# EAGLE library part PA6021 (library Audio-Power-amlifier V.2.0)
The PA6021 is a stereo audio power amplifier that drives 2 W/channel of continuous RMS power into a 4-Ω load when utilizing a heat sink. Advanced dc volume control minimizes external components and allows BTL (speaker) volume control and SE (headphone) volume control.
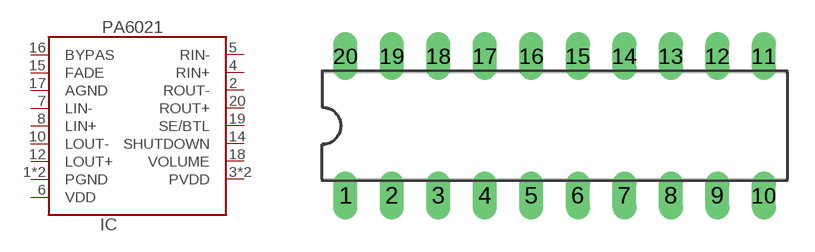
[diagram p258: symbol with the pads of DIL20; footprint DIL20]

Designator prefix IC

## PA6021  [DIL20]
1  PGND  pwr
2  ROUT-  out
3  PVDD  pwr
4  RIN+  in
5  RIN-  in
6  VDD  pwr
7  LIN-  in
8  LIN+  in
9  PVDD  pwr
10  LOUT-  out
11  PGND  pwr
12  LOUT+  out
14  SHUTDOWN  in
15  FADE  in
16  BYPAS  in
17  AGND  pwr
18  VOLUME  in
19  SE/BTL  in
20  ROUT+  out

## Footprint DIL20 (pad centres in mm)
Dual In Line Package
drill 0.813 long: 1 -11.43,-3.81; 2 -8.89,-3.81; 3 -6.35,-3.81; 4 -3.81,-3.81; 5 -1.27,-3.81; 6 1.27,-3.81; 7 3.81,-3.81; 8 6.35,-3.81; 9 8.89,-3.81; 10 11.43,-3.81; 11 11.43,3.81; 12 8.89,3.81; 13 6.35,3.81; 14 3.81,3.81; 15 1.27,3.81; 16 -1.27,3.81; 17 -3.81,3.81; 18 -6.35,3.81; 19 -8.89,3.81; 20 -11.43,3.81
